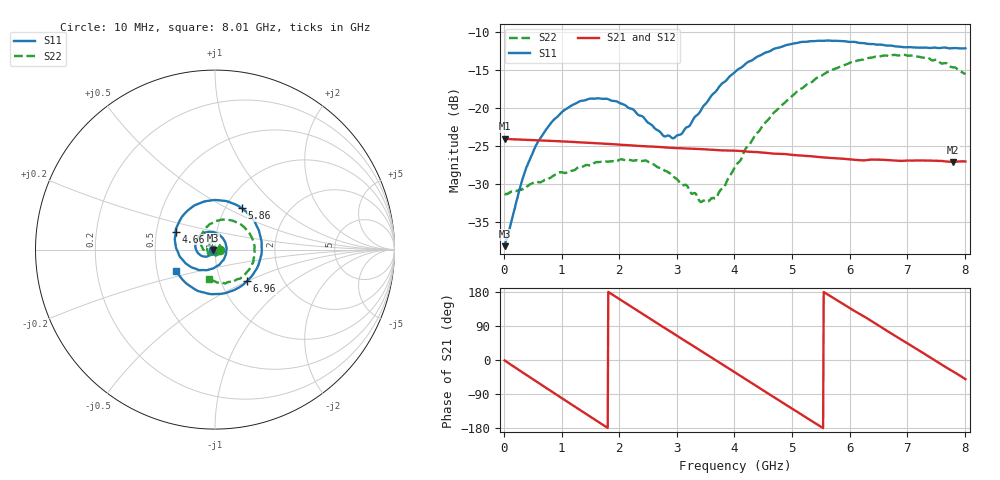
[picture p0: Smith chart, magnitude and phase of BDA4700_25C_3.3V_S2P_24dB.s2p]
!Agilent Technologies,E5071B,MY42404982,A.09.10
!Date: Mon Oct 20 18:13:09 2025
!Data & Calibration Information:
!Freq	S11:SOLT2(ON)	S21:SOLT2(ON)	S12:SOLT2(ON)	S22:SOLT2(ON)
# Hz S RI R 50
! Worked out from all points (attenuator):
!   801 points, 10 MHz to 8.01 GHz, reference 50 ohm
!   highest |S21| = -24.06 dB at 10 MHz (marker M1); lowest = -27.1 dB at 7.8 GHz (marker M2)
!   lowest |S11| = -38.2 dB at 10 MHz (marker M3), VSWR 1.02, Z = 48.8 - j0.15 ohm
!   |S11| at or under -10 dB: start of sweep to end of sweep
!   |S22| runs from -32.4 to -13.0 dB; largest |S21 - S12| = 0.00069
!   S11 on the Smith chart (normalised r, x): 10 MHz: 0.98, -0.00; 4.66 GHz: 0.63, +0.13; 5.86 GHz: 1.19, +0.59; 6.96 GHz: 1.33, -0.50; 8.01 GHz: 0.63, -0.16
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1e7  -0.0122 -0.00154  0.0626 -0.00134  0.0626 -0.0014  0.0271 -0.000803
3.4e8  -0.0235 -0.0271  0.0508 -0.035  0.0508 -0.035  0.0233 -0.018
5.7e8  -0.0432 -0.0387  0.0329 -0.0516  0.0328 -0.0517  0.0148 -0.0291
8.7e8  -0.0765 -0.0341  0.00271 -0.0605  0.0027 -0.0604  -0.00633 -0.0355
1.35e9  -0.1098 0.0191  -0.0419 -0.0419  -0.0419 -0.0419  -0.0366 -0.0182
1.96e9  -0.0555 0.0951  -0.0554 0.0149  -0.0555 0.0149  -0.0352 0.0273
2.45e9  0.0278 0.0793  -0.0256 0.0496  -0.0256 0.0496  -0.00305 0.045
2.68e9  0.056 0.0435  -0.00486 0.0551  -0.00496 0.055  0.0132 0.0383
2.96e9  0.062 -0.0141  0.0202 0.0505  0.0202 0.0504  0.0263 0.023
3.43e9  0.000962 -0.0983  0.0492 0.0209  0.0493 0.021  0.0201 -0.0132
3.69e9  -0.0626 -0.114  0.0528 -0.00176  0.0528 -0.0019  0.00135 -0.0258
4.01e9  -0.1479 -0.0877  0.0439 -0.0283  0.0439 -0.0282  -0.0314 -0.0262
4.66e9  -0.2193 0.1005  -0.00492 -0.0498  -0.00477 -0.0499  -0.0796 0.0438
4.98e9  -0.1683 0.2016  -0.0292 -0.0396  -0.0291 -0.0398  -0.0672 0.0966
5.35e9  -0.0467 0.2705  -0.0455 -0.0151  -0.0454 -0.0153  -0.016 0.1473
5.86e9  0.1494 0.2307  -0.0402 0.0229  -0.0401 0.0229  0.098 0.1611
6.27e9  0.2473 0.0964  -0.0179 0.0415  -0.0172 0.0418  0.1835 0.1016
6.68e9  0.2452 -0.0758  0.0125 0.0435  0.0126 0.0436  0.2201 -0.000187
6.96e9  0.1788 -0.1748  0.0298 0.0336  0.03 0.0334  0.2099 -0.0757
7.39e9  0.00996 -0.2475  0.0446 0.00602  0.0446 0.00603  0.133 -0.1631
7.8e9  -0.1576 -0.1904  0.038 -0.0224  0.038 -0.0226  0.0194 -0.1836
8.01e9  -0.2148 -0.1215  0.0282 -0.0343  0.0284 -0.0342  -0.031 -0.1634
